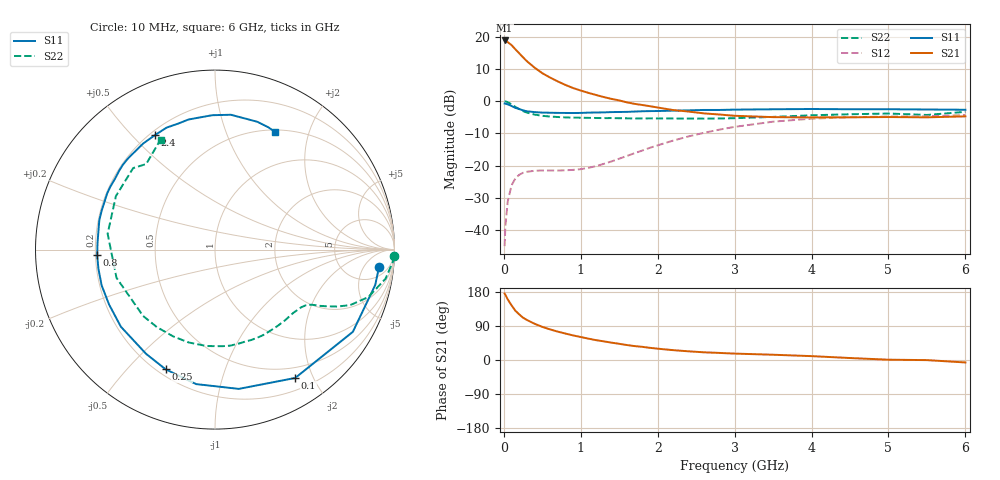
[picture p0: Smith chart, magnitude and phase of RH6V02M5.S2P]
! SIEMENS Small Signal Semiconductors
! BFR106
! Si NPN RF Bipolar Junction Transistor in SOT23
! VCE = 6 V  IC = 2.5 mA
! Common Emitter S-Parameters:  August  1996
# GHz  S  MA  R  50
!  f  S11  S21  S12  S22
! GHz  MAG  ANG  MAG  ANG  MAG  ANG  MAG  ANG
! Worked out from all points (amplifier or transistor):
!   36 points, 10 MHz to 6 GHz, reference 50 ohm
!   highest |S21| = 18.8 dB at 10 MHz (marker M1)
!   |S21| within 3 dB of that: start of sweep to 160.7 MHz
!   unconditionally stable (mu >= 1): 750.6 MHz to 1.825 GHz; 4.315 GHz to end of sweep
!   at 250 MHz: K = 0.35, MSG = 17.9 dB, |S12| = -22.2 dB
!   at 1.4 GHz: K = 1.20, MAG = 6.9 dB, |S12| = -18.7 dB
!   at 6 GHz: K = 1.02, MAG = -1.1 dB, |S12| = -4.3 dB
!   S11 on the Smith chart (normalised r, x): 10 MHz: 9, -11; 100 MHz: 0.35, -1.75; 250 MHz: 0.23, -0.64; 800 MHz: 0.21, -0.02; 2.4 GHz: 0.22, +0.58; 6 GHz: 0.52, +1.50
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0.01  0.919 -6.2  8.701 175.3  0.0057 87.4  0.9989 -2.1
0.02  0.9141 -12.5  8.614 172.1  0.0116 84.0  0.9923 -4.1
0.05  0.8943 -30.8  8.197 160.1  0.0278 73.5  0.9637 -9.7
0.1  0.8433 -58.0  7.378 144.3  0.0498 60.5  0.8945 -17.2
0.15  0.7873 -80.3  6.35 130.0  0.0638 49.6  0.8145 -22.3
0.2  0.7567 -98.0  5.508 120.3  0.0726 43.0  0.7534 -24.9
0.25  0.7214 -112.4  4.763 111.6  0.078 37.7  0.7007 -26.8
0.3  0.6964 -123.4  4.151 105.6  0.0807 34.7  0.6662 -28.1
0.4  0.6779 -140.7  3.3 95.6  0.0838 31.2  0.6197 -29.7
0.5  0.6648 -152.7  2.71 87.4  0.0846 30.1  0.5934 -31.5
0.6  0.6623 -162.5  2.323 80.8  0.0846 31.2  0.5785 -33.7
0.8  0.6571 -177.2  1.783 69.8  0.0851 36.8  0.5606 -39.1
1.1  0.6651 165.7  1.344 56.4  0.093 50.8  0.5512 -48.8
1.6  0.6827 144.7  0.958 39.5  0.142 68.1  0.5427 -67.9
2.2  0.7139 124.0  0.729 26.0  0.2453 68.7  0.5394 -95.0
2.4  0.7204 117.6  0.691 22.9  0.2846 65.9  0.5378 -105.7
3  0.7398 101.5  0.594 16.9  0.4003 54.0  0.5451 -137.3
3.5  0.749 91.1  0.566 13.9  0.4816 42.3  0.5708 -164.0
4.5  0.7493 77.1  0.563 5.2  0.5641 20.0  0.6275 151.6
5  0.7502 71.7  0.568 0.8  0.5789 11.2  0.6436 135.1
5.5  0.7431 66.3  0.562 -0.3  0.5821 6.9  0.6118 128.8
6  0.7364 63.2  0.582 -6.5  0.6104 -1.3  0.6839 116.3
